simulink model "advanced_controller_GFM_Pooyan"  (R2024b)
settings: Solver=VariableStepAuto  StartTime=0.0  StopTime=2  RelTol=1e-3
model workspace (MAT data in the model file):
  b1 = 1000.38104695
  b2 = 1006.47399607
  b3 = 1006.95432939
  b4 = 996.322108769
  b5 = 995.669039411
  b6 = 1012.96535236
  b7 = 1007.5422409
  b8 = 993.960341463
  l1 = 8282.83466164
  l10 = 5511.54621883
  l11 = 8516.9845943
  l12 = 3533.51403234
  l13 = 1255.67117866
  l14 = 1105.23671469
  l15 = 955.492069576
  l16 = 1255.83166019
  l2 = 7767.51754481
  l3 = 6680.69860842
  l4 = 3013.93364227
  l5 = 912.604633733
  l6 = 706.803488619
  l7 = 1117.39027011
  l8 = 1674.30810947
  l9 = 1971.00014576
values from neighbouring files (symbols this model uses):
  alpha_p = 0.0001    [initialcondition_Pooyan.m]    (also in initialcondition_gfm_Pooyan.m = 0.0005)
  alpha_q = 0.0001    [initialcondition_Pooyan.m]    (also in initialcondition_gfm_Pooyan.m)
  Cf = 50e-6    (= 5e-05)    [initialcondition_Pooyan.m]    (also in initialcondition_gfm_Pooyan.m)
  Kicc = 314.159    [initialcondition_Pooyan.m]    (also in initialcondition_gfm_Pooyan.m)
  Kivc = 400    [initialcondition_Pooyan.m]    (also in initialcondition_gfm_Pooyan.m)
  Kpcc = 31.4159    [initialcondition_Pooyan.m]    (also in initialcondition_gfm_Pooyan.m)
  Kpvc = 0.5    [initialcondition_Pooyan.m]    (also in initialcondition_gfm_Pooyan.m)
  Lf = 10e-3    (= 0.01)    [initialcondition_Pooyan.m]    (also in initialcondition_gfm_Pooyan.m)
  Lg = X_BY_R*Rg/(wn)    [initialcondition_Pooyan.m]    (also in initialcondition_gfm_Pooyan.m; DER_param.m = (X_BY_R_gfl * Rg) / wn_gfl)
  Pn = 20e3    (= 20000)    [initialcondition_Pooyan.m]    (also in initialcondition_gfm_Pooyan.m)
  Qn = 0    [initialcondition_Pooyan.m]    (also in initialcondition_gfm_Pooyan.m)
  R = (3*Vg^2)/(2*Pn)    (= 8.000067)    [initialcondition_Pooyan.m]    (also in MC2.m = (8760*SS-sum(Tdown))/(8760*SS); initialcondition_gfm_Pooyan.m)
  Rf = 0.1    [initialcondition_Pooyan.m]    (also in initialcondition_gfm_Pooyan.m)
  Rg = (3*Vg^2)/(2*SCR*sqrt(1+X_BY_R^2)*Pn)    [initialcondition_Pooyan.m]    (also in initialcondition_gfm_Pooyan.m; DER_param.m = (3 * Vg_gfl^2) / (2 * SCR_gfl * sqrt(1 + X_BY_R_gfl^2) * Pn_)
  tau_p = 0.031415    [initialcondition_Pooyan.m]    (also in initialcondition_gfm_Pooyan.m)
  tau_q = 0.031415    [initialcondition_Pooyan.m]    (also in initialcondition_gfm_Pooyan.m)
  Ts = 50e-6    (= 5e-05)    [initialcondition_Pooyan.m]    (also in initialcondition_gfm_Pooyan.m)
  Vdc = 700    [initialcondition_Pooyan.m]    (also in initialcondition_gfm_Pooyan.m)
  Vg = 326.6    [initialcondition_Pooyan.m]    (also in initialcondition_gfm_Pooyan.m)
  wn = 2*pi*50    (= 314.159265359)    [initialcondition_Pooyan.m]    (also in initialcondition_gfm_Pooyan.m)
undefined symbols (not defined in the file or in its folder): DiscIntNeverNeededParam
libraries: simulink x8, spsThreePhaseSeriesRLCBranchLib x4, spsThreePhaseVIMeasurementLib x3, spsabctodq0Lib x3, spsGroundLib x2, spsDCVoltageSourceLib x1, spsThreePhaseSourceLib x1, spsThreePhaseBreakerLib x1, spsUniversalBridgeLib x1, spsdq0toabcLib x1, sps_lib x1

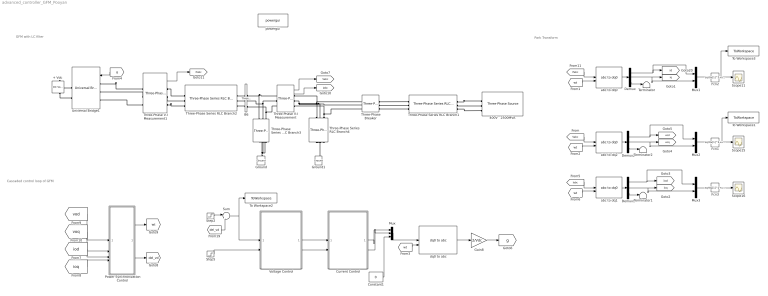
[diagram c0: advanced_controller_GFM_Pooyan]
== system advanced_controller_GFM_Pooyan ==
  note: Cascaded control loop of GFM
  note: GFM with LC filter
  note: Park Transform
  "+ Vdc " : spsDCVoltageSourceLib/DC Voltage Source  Amplitude=Vdc  Measurements=None
  400V   2500MVA : spsThreePhaseSourceLib/Three-Phase Source  InternalConnection=Yg  VoltagePhases=off  Voltage=Vg*sqrt(3/2)  PhaseAngle=0  Voltage_phases=[25e3 25e3 25e3]/sqrt(3)  PhaseAngles_phases=[0 -120 +120]  Frequency=50  NonIdealSource=on  SpecifyImpedance=off  Resistance=0  Inductance=0  ShortCircuitLevel=2500e6  BaseVoltage=Vg*sqrt(3/2)  XRratio=7  BusType=swing  Pref=0  Qref=0  Prefabc=[10e3, 10e3, 10e3]  Qrefabc=[0, 0, 0]  Qmin=-inf  Qmax=inf
  B6 : spsThreePhaseVIMeasurementLib/Three-Phase V-I Measurement  VoltageMeasurement=phase-to-ground  SetLabelV=on  LabelV=Vabcg  Vpu=on  VpuLL=off  CurrentMeasurement=yes  SetLabelI=on  LabelI=Iabcg  Ipu=off  Pbase=100e3  Vbase=415  OutputType=Magnitude  PhasorSimulation=off  PSBequivalent=0
  Constant1 : Constant  Value=0
  Current Control : Subsystem
  Demux : Demux  Outputs=3
  Demux1 : Demux  Outputs=3
  Demux2 : Demux  Outputs=3
  Fcn1 : Fcn  Expr=sqrt(u[1]^2+u[2]^2)
  Fcn2 : Fcn  Expr=sqrt(u[1]^2+u[2]^2)
  Fcn3 : Fcn  Expr=sqrt(u[1]^2+u[2]^2)
  Gain8 : Gain  Gain=2/Vdc
  Ground : spsGroundLib/Ground  LConnTagsString=a
  Ground1 : spsGroundLib/Ground  LConnTagsString=a
  Mux : Mux  Inputs=3
  Mux1 : Mux  Inputs=2
  Mux2 : Mux  Inputs=2
  Mux3 : Mux  Inputs=2
  Power Synchronization Control : Subsystem
  Scope11 : Scope
  Scope15 : Scope
  Scope16 : Scope
  Step2 : Step  Time=100  Before=Vg  After=Vg  SampleTime=0
  Step5 : Step  Time=100  After=0  SampleTime=0
  Sum : Sum  Inputs=|++
  Terminator : Terminator
  Terminator1 : Terminator
  Terminator2 : Terminator
  Three-Phase Series RLC Branch1 : spsThreePhaseSeriesRLCBranchLib/Three-Phase Series RLC Branch  LConnTagsString=A|B|C  RConnTagsString=A|B|C  BranchType=RL  Resistance=Rg  Inductance=Lg  Capacitance=1e-6  Measurements=None
  Three-Phase Series RLC Branch2 : spsThreePhaseSeriesRLCBranchLib/Three-Phase Series RLC Branch  LConnTagsString=A|B|C  RConnTagsString=A|B|C  BranchType=RL  Resistance=Rf  Inductance=Lf  Capacitance=1e-6  Measurements=None
  Three-Phase Series RLC Branch3 : spsThreePhaseSeriesRLCBranchLib/Three-Phase Series RLC Branch  LConnTagsString=A|B|C  RConnTagsString=A|B|C  BranchType=C  Resistance=0.1  Inductance=280e-3  Capacitance=Cf  Measurements=None
  Three-Phase Series RLC Branch4 : spsThreePhaseSeriesRLCBranchLib/Three-Phase Series RLC Branch  LConnTagsString=A|B|C  RConnTagsString=A|B|C  BranchType=R  Resistance=R  Inductance=0  Capacitance=1e-6  Measurements=None
  Three-Phase V-I Measurement : spsThreePhaseVIMeasurementLib/Three-Phase V-I Measurement  VoltageMeasurement=phase-to-ground  SetLabelV=off  LabelV=Vabc  Vpu=off  VpuLL=off  CurrentMeasurement=yes  SetLabelI=off  LabelI=Iabc  Ipu=off  Pbase=100e6  Vbase=500e3  OutputType=Complex  PhasorSimulation=off  PSBequivalent=0
  Three-Phase V-I Measurement1 : spsThreePhaseVIMeasurementLib/Three-Phase V-I Measurement  VoltageMeasurement=no  SetLabelV=off  LabelV=Vabc  Vpu=off  VpuLL=off  CurrentMeasurement=yes  SetLabelI=off  LabelI=Iabc  Ipu=off  Pbase=100e6  Vbase=500e3  OutputType=Complex  PhasorSimulation=off  PSBequivalent=0
  Three-Phase Breaker : spsThreePhaseBreakerLib/Three-Phase Breaker  InitialState=open  SwitchA=on  SwitchB=on  SwitchC=on  SwitchTimes=[0.5]  External=off  BreakerResistance=0.01  SnubberResistance=1e6  SnubberCapacitance=inf  Measurements=None
  To Workspace1 : ToWorkspace  VariableName=vo2  SampleTime=-1
  To Workspace2 : ToWorkspace  VariableName=vd_ref  SampleTime=-1
  To Workspace3 : ToWorkspace  VariableName=if2  SampleTime=-1
  Universal Bridge1 : spsUniversalBridgeLib/Universal Bridge  Arms=3  SnubberResistance=1e5  SnubberCapacitance=inf  Device=Average-model based VSC  Ron=1e-3  Lon=0  ForwardVoltages="[  0  0  ]"  ForwardVoltage=0  GTOparameters=[ 10e-6 , 20e-6 ]  IGBTparameters=[ 1e-6 , 2e-6 ]  Measurements=None  Measurements_2=None  converterType=Rectifier
  Voltage Control : Subsystem
  abc to dq0 : spsabctodq0Lib/abc to dq0  Alignment=90 degrees behind phase A axis
  abc to dq1 : spsabctodq0Lib/abc to dq0  Alignment=90 degrees behind phase A axis
  abc to dq2 : spsabctodq0Lib/abc to dq0  Alignment=90 degrees behind phase A axis
  dq0 to abc : spsdq0toabcLib/dq0 to abc  Alignment=90 degrees behind phase A axis
  powergui : sps_lib/powergui  Priority=1  SimulationMode=Discrete  SampleTime=Ts  frequency=50  Iterations=50  frequencyindice=0  Pbase=100e6  ErrMax=1e-4  UnitsV=kV  UnitsW=MW  buscounter=0  FunctionMessages=off  echomessages=off  EnableUseOfTLC=off  CurrentSourceSwitches=off  DisableSnubberDevices=off  DisableRonSwitches=off  DisableVfSwitches=off  DisplayEquations=off  AutomaticDiscreteSolvers=off  SolverType=Tustin  Interpol=off  ExternalGateDelay=off  methode=off  Ts=0  x0status=blocks  SPID=off  SwTol=0  HookPort=off  NonlinearTolerance=0  nMaxIteration=15  ContinueOnMaxIteration=off  RestoreLinks=warning  ResistiveCurrentMeasurement=off  Frange=[0:2:500]  Ylog=off  Xlog=on  ShowGrid=off  save=off  variable=ZData  structure=0  ZoomFFT=on  StartTime=0.0  cycles=1  DisplayStyle=1  fundamental=60  FreqAxis=off  MaxFrequency=1000  frequencyindicesteady=1  RmsSteady=1  display=off
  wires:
  Gain8/1 -> [g]
  Demux/3 -> Terminator/1
  abc to dq1/1 -> Demux1/1
  Step2/1 -> Sum/1
  [wt] -> dq0 to abc/2
  Constant1/1 -> Mux/3
  [ioq] -> Power Synchronization Control/4(In4)
  [iod] -> Power Synchronization Control/3(In3)
  dq0 to abc/1 -> Gain8/1
  Demux/2 -> Mux1/2, [iq]
  Mux/1 -> dq0 to abc/1
  [wt] -> abc to dq2/2
  [vod] -> Power Synchronization Control/1(In1)
  Demux1/3 -> Terminator1/1
  Demux1/2 -> Mux3/2, [ioq]
  Voltage Control/2(iqref) -> Current Control/2(iqref)
  Current Control/2(vqt) -> Mux/2
  [voq] -> Power Synchronization Control/2(In2)
  Demux1/1 -> Mux3/1, [iod]
  Demux2/1 -> Mux2/1, [vod]
  [g] -> Universal Bridge1/1
  [del_vd] -> Sum/2
  Voltage Control/1(idref) -> Current Control/1(idref)
  [wt] -> abc to dq0/2
  Demux/1 -> Mux1/1, [id]
  abc to dq2/1 -> Demux2/1
  Current Control/1(vdt) -> Mux/1
  Demux2/3 -> Terminator2/1
  Power Synchronization Control/2(del_vd) -> [del_vd]
  Sum/1 -> Voltage Control/1(vodref), To Workspace2/1
  Power Synchronization Control/1(wt) -> [wt]
  Demux2/2 -> [voq], Mux2/2
  abc to dq0/1 -> Demux/1
  Mux1/1 -> Fcn2/1
  Fcn2/1 -> To Workspace3/1, Scope11/1
  Mux2/1 -> Fcn1/1
  Fcn1/1 -> To Workspace1/1, Scope15/1
  Fcn3/1 -> Scope16/1
  Mux3/1 -> Fcn3/1
  Three-Phase V-I Measurement/1 -> [Vabc]
  [Vabc] -> abc to dq2/1
  Three-Phase V-I Measurement/2 -> [Iabc]
  [Iabc] -> abc to dq1/1
  [wt] -> abc to dq1/2
  Three-Phase V-I Measurement1/1 -> [Ifabc]
  [Ifabc] -> abc to dq0/1
  Step5/1 -> Voltage Control/2(voqref)
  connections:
  Three-Phase Series RLC Branch3/LConn3 -- Three-Phase V-I Measurement/LConn3 -- B6/RConn3
  Three-Phase Series RLC Branch4/LConn1 -- Three-Phase Breaker/LConn1 -- Three-Phase V-I Measurement/RConn1
  Three-Phase Series RLC Branch3/LConn1 -- Three-Phase V-I Measurement/LConn1 -- B6/RConn1
  Three-Phase Series RLC Branch4/RConn3 -- Three-Phase Series RLC Branch4/RConn1 -- Ground1/LConn1 -- Three-Phase Series RLC Branch4/RConn2
  Three-Phase V-I Measurement/RConn2 -- Three-Phase Breaker/LConn2 -- Three-Phase Series RLC Branch4/LConn2
  Three-Phase Series RLC Branch3/LConn2 -- B6/RConn2 -- Three-Phase V-I Measurement/LConn2
  Ground/LConn1 -- Three-Phase Series RLC Branch3/RConn1 -- Three-Phase Series RLC Branch3/RConn2 -- Three-Phase Series RLC Branch3/RConn3
  Three-Phase Series RLC Branch4/LConn3 -- Three-Phase Breaker/LConn3 -- Three-Phase V-I Measurement/RConn3
  Three-Phase V-I Measurement1/LConn3 -- Universal Bridge1/LConn3
  Three-Phase V-I Measurement1/LConn2 -- Universal Bridge1/LConn2
  Three-Phase Breaker/RConn1 -- Three-Phase Series RLC Branch1/LConn1
  Three-Phase Breaker/RConn3 -- Three-Phase Series RLC Branch1/LConn3
  Three-Phase Series RLC Branch1/RConn1 -- 400V   2500MVA/RConn1
  Three-Phase V-I Measurement1/RConn1 -- Three-Phase Series RLC Branch2/LConn1
  "+ Vdc "/RConn1 -- Universal Bridge1/RConn1
  Three-Phase Series RLC Branch1/RConn2 -- 400V   2500MVA/RConn2
  Three-Phase Series RLC Branch1/RConn3 -- 400V   2500MVA/RConn3
  "+ Vdc "/LConn1 -- Universal Bridge1/RConn2
  Three-Phase Breaker/RConn2 -- Three-Phase Series RLC Branch1/LConn2
  Three-Phase V-I Measurement1/RConn2 -- Three-Phase Series RLC Branch2/LConn2
  Universal Bridge1/LConn1 -- Three-Phase V-I Measurement1/LConn1
  B6/LConn3 -- Three-Phase Series RLC Branch2/RConn3
  B6/LConn2 -- Three-Phase Series RLC Branch2/RConn2
  Three-Phase V-I Measurement1/RConn3 -- Three-Phase Series RLC Branch2/LConn3
  B6/LConn1 -- Three-Phase Series RLC Branch2/RConn1

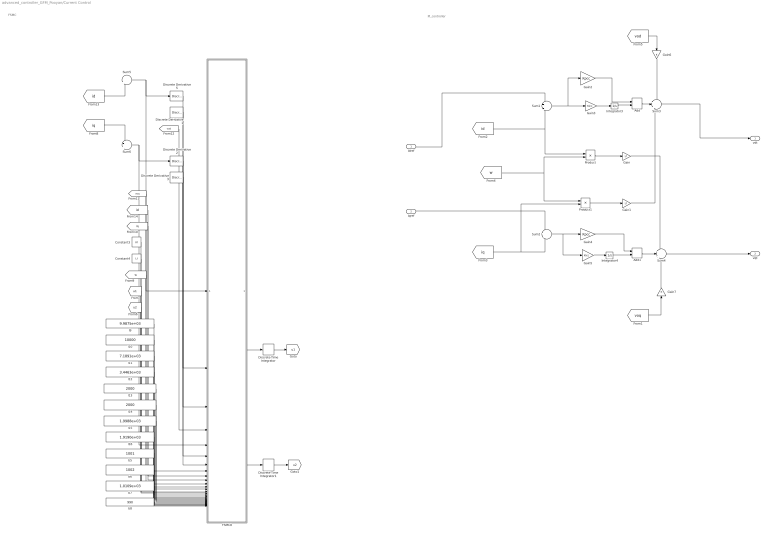
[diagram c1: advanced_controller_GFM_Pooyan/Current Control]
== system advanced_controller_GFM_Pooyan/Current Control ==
  note: PI_controller
  note: FSMC
  idref : Inport
  iqref : Inport  Port=2
  Add : Sum
  Add1 : Sum
  Constant3 : Constant  Commented=on  Value=Rf
  Constant4 : Constant  Commented=on  Value=Lf
  Discrete Derivative{1..3,5} (4 alike) : simulink/Quick Insert/Discrete/Discrete Derivative  Commented=on  gainval=1.0  ICPrevScaledInput=0.0  OutMin=[]  OutMax=[]  OutDataType=fixdt(1, 16)  OutScaling=2^-10  DoSatur=off
  Discrete-Time Integrator : DiscreteIntegrator  Commented=on  SampleTime=-1  ICPrevOutput=DiscIntNeverNeededParam  ICPrevScaledInput=DiscIntNeverNeededParam
  Discrete-Time Integrator1 : DiscreteIntegrator  Commented=on  SampleTime=-1  ICPrevOutput=DiscIntNeverNeededParam  ICPrevScaledInput=DiscIntNeverNeededParam
  FSMC8 : MATLAB Function  Commented=on  TreatAsAtomicUnit=on
  Gain : Gain  Gain=Lf
  Gain1 : Gain  Gain=Lf
  Gain2 : Gain  Gain=Kpcc
  Gain3 : Gain  Gain=Kicc
  Gain4 : Gain  Gain=Kpcc
  Gain5 : Gain  Gain=Kicc
  Gain6 : Gain
  Gain7 : Gain
  Integrator3 : Integrator
  Integrator4 : Integrator
  Product : Product
  Product1 : Product
  Sum1 : Sum  Inputs=+|-
  Sum2 : Sum  Inputs=+|-
  Sum3 : Sum  Inputs=+|+|-
  Sum4 : Sum  Inputs=+|+|+
  Sum5 : Sum  Commented=on  Inputs=|+-
  Sum6 : Sum  Commented=on  Inputs=-+|
  b5 : Constant  Commented=on  Value=1001
  b6 : Constant  Commented=on  Value=1002
  b7 : Constant  Commented=on  Value=1.0109e+03
  b8 : Constant  Commented=on  Value=990
  l10 : Constant  Commented=on  Value=10000
  l11 : Constant  Commented=on  Value=7.1891e+03
  l12 : Constant  Commented=on  Value=3.4463e+03
  l13 : Constant  Commented=on  Value=2000
  l14 : Constant  Commented=on  Value=2000
  l15 : Constant  Commented=on  Value=1.9988e+03
  l16 : Constant  Commented=on  Value=1.9190e+03
  l9 : Constant  Commented=on  Value=9.9875e+03
  vdt : Outport
  vqt : Outport  Port=2
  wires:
  Gain3/1 -> Integrator3/1
  Integrator4/1 -> Add1/2
  Add/1 -> Sum3/2
  Gain4/1 -> Add1/1
  Add1/1 -> Sum4/2
  Gain2/1 -> Add/1
  Gain/1 -> Sum4/1
  Gain1/1 -> Sum3/3
  Integrator3/1 -> Add/2
  Gain5/1 -> Integrator4/1
  iqref/1 -> Sum2/1
  [iq] -> Sum2/2, Product1/2
  idref/1 -> Sum1/1
  [id] -> Product/1, Sum1/2
  Product/1 -> Gain/1
  Product1/1 -> Gain1/1
  [w] -> Product1/1, Product/2
  [vod] -> Gain6/1
  [voq] -> Gain7/1
  Gain6/1 -> Sum3/1
  Gain7/1 -> Sum4/3
  Sum3/1 -> vdt/1
  Sum4/1 -> vqt/1
  Constant4/1 -> FSMC8/12(Lf)
  l10/1 -> FSMC8/17(a_2)
  Discrete Derivative2/1 -> FSMC8/6(e2dot)
  b7/1 -> FSMC8/26(betta2s)
  FSMC8/2(vqt) -> ?
  FSMC8/3(u1dot) -> Discrete-Time Integrator/1
  Discrete Derivative5/1 -> FSMC8/2(e1dot)
  [w] -> FSMC8/13(w)
  Sum6/1 -> FSMC8/5(e2), Discrete Derivative2/1
  Sum5/1 -> FSMC8/1(e1), Discrete Derivative5/1
  [voq] -> FSMC8/8(voq)
  Constant3/1 -> FSMC8/11(Rf)
  l16/1 -> FSMC8/23(a_8)
  [iq] -> FSMC8/10(ioq)
  l13/1 -> FSMC8/20(a_5)
  l11/1 -> FSMC8/18(a_3)
  [id] -> Sum5/2
  FSMC8/1(vdt) -> ?
  b6/1 -> FSMC8/25(betta1m)
  l12/1 -> FSMC8/19(a_4)
  l14/1 -> FSMC8/21(a_6)
  Discrete Derivative3/1 -> FSMC8/7(iqrefdot)
  b5/1 -> FSMC8/24(betta1s)
  l9/1 -> FSMC8/16(a_1)
  b8/1 -> FSMC8/27(betta2m)
  [id] -> FSMC8/9(iod)
  Discrete Derivative1/1 -> FSMC8/3(idrefdot)
  FSMC8/4(u2dot) -> Discrete-Time Integrator1/1
  ? -> Discrete Derivative1/1, Sum5/1
  [vod] -> FSMC8/4(vod)
  [iq] -> Sum6/1
  ? -> Discrete Derivative3/1, Sum6/2
  l15/1 -> FSMC8/22(a_7)
  Sum1/1 -> Gain3/1, Gain2/1
  Sum2/1 -> Gain5/1, Gain4/1
  Discrete-Time Integrator/1 -> [u1]
  Discrete-Time Integrator1/1 -> [u2]
  [u1] -> FSMC8/14(u1)
  [u2] -> FSMC8/15(u2)

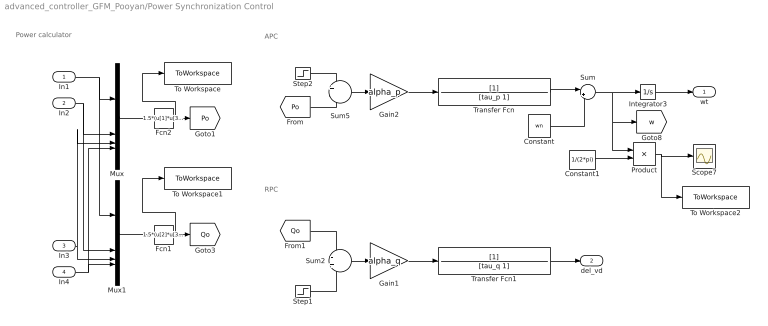
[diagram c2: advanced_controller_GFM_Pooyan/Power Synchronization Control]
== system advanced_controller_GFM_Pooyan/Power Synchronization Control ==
  note: APC
  note: RPC
  note: Power calculator
  In1 : Inport
  In2 : Inport  Port=2
  In3 : Inport  Port=3
  In4 : Inport  Port=4
  Constant : Constant  Value=wn
  Constant1 : Constant  Value=1/(2*pi)
  Fcn1 : Fcn  Expr=1.5*(u[2]*u[3]-u[1]*u[4])
  Fcn2 : Fcn  Expr=1.5*(u[1]*u[3]+u[2]*u[4])
  Gain1 : Gain  Gain=alpha_q
  Gain2 : Gain  Gain=alpha_p
  Integrator3 : Integrator
  Mux : Mux
  Mux1 : Mux
  Product : Product
  Scope7 : Scope
  Step1 : Step  Time=100  Before=Qn  After=Qn  SampleTime=0
  Step2 : Step  Time=100  Before=Pn  After=Pn  SampleTime=0
  Sum : Sum  Inputs=|++
  Sum2 : Sum  Inputs=-+
  Sum5 : Sum  Inputs=+-
  To Workspace : ToWorkspace  VariableName=Po  SampleTime=-1
  To Workspace1 : ToWorkspace  VariableName=Qo  SampleTime=-1
  To Workspace2 : ToWorkspace  VariableName=f  SampleTime=-1
  Transfer Fcn : TransferFcn  Denominator=[tau_p 1]  ParameterTunability=Unconstrained
  Transfer Fcn1 : TransferFcn  Denominator=[tau_q 1]  ParameterTunability=Unconstrained
  wt : Outport
  del_vd : Outport  Port=2
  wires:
  Sum5/1 -> Gain2/1
  [Po] -> Sum5/2
  Fcn2/1 -> To Workspace/1, [Po]
  [Qo] -> Sum2/1
  Step1/1 -> Sum2/2
  Sum2/1 -> Gain1/1
  Step2/1 -> Sum5/1
  Gain1/1 -> Transfer Fcn1/1
  Transfer Fcn1/1 -> del_vd/1
  Gain2/1 -> Transfer Fcn/1
  Transfer Fcn/1 -> Sum/1
  Constant/1 -> Sum/2
  Sum/1 -> [w], Product/1, Integrator3/1
  Mux/1 -> Fcn2/1
  Constant1/1 -> Product/2
  Integrator3/1 -> wt/1
  Product/1 -> To Workspace2/1, Scope7/1
  In3/1 -> Mux1/3, Mux/3
  In1/1 -> Mux1/1, Mux/1
  In4/1 -> Mux/4, Mux1/4
  In2/1 -> Mux1/2, Mux/2
  Mux1/1 -> Fcn1/1
  Fcn1/1 -> To Workspace1/1, [Qo]

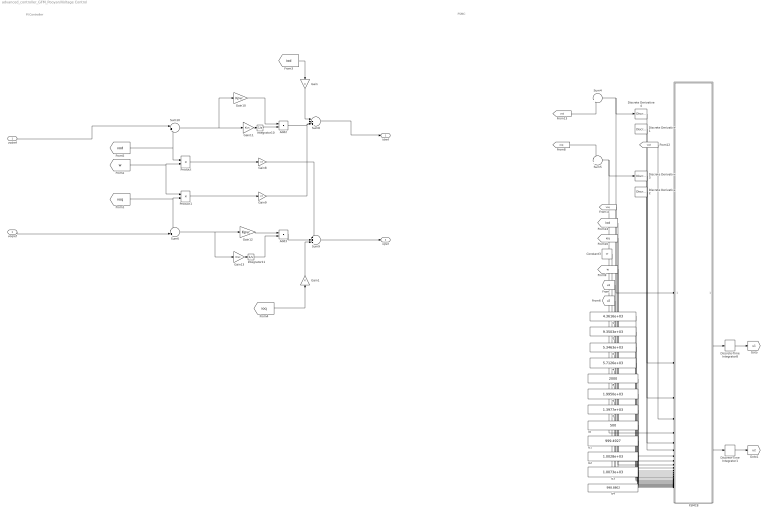
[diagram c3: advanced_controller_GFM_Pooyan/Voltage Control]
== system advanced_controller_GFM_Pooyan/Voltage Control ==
  note: PI Controller
  note: FSMC
  vodref : Inport
  voqref : Inport  Port=2
  Add2 : Sum
  Add3 : Sum
  Constant3 : Constant  Commented=on  Value=Cf
  Discrete Derivative{1..4} (4 alike) : simulink/Quick Insert/Discrete/Discrete Derivative  Commented=on  gainval=1.0  ICPrevScaledInput=0.0  OutMin=[]  OutMax=[]  OutDataType=fixdt(1, 16)  OutScaling=2^-10  DoSatur=off
  Discrete-Time Integrator1 : DiscreteIntegrator  Commented=on  SampleTime=-1  ICPrevOutput=DiscIntNeverNeededParam  ICPrevScaledInput=DiscIntNeverNeededParam
  Discrete-Time Integrator8 : DiscreteIntegrator  Commented=on  SampleTime=-1  ICPrevOutput=DiscIntNeverNeededParam  ICPrevScaledInput=DiscIntNeverNeededParam
  FSMC8 : MATLAB Function  Commented=on  TreatAsAtomicUnit=on
  Gain : Gain
  Gain1 : Gain
  Gain10 : Gain  Gain=Kpvc
  Gain11 : Gain  Gain=Kivc
  Gain12 : Gain  Gain=Kpvc
  Gain13 : Gain  Gain=Kivc
  Gain8 : Gain  Gain=Cf
  Gain9 : Gain  Gain=Cf
  Integrator10 : Integrator
  Integrator11 : Integrator
  Product : Product
  Product1 : Product
  Sum10 : Sum  Inputs=|+-
  Sum4 : Sum  Commented=on  Inputs=|+-
  Sum5 : Sum  Commented=on  Inputs=-+|
  Sum6 : Sum  Inputs=-+|
  Sum8 : Sum  Inputs=|++-
  Sum9 : Sum  Inputs=+++|
  b1 : Constant  Commented=on  Value=999.4927
  b2 : Constant  Commented=on  Value=1.0028e+03
  b3 : Constant  Commented=on  Value=1.0073e+03
  b4 : Constant  Commented=on  Value=998.8802
  l1 : Constant  Commented=on  Value=4.3616e+03
  l2 : Constant  Commented=on  Value=9.3503e+03
  l3 : Constant  Commented=on  Value=5.3463e+03
  l4 : Constant  Commented=on  Value=5.7126e+03
  l5 : Constant  Commented=on  Value=2000
  l6 : Constant  Commented=on  Value=1.9950e+03
  l7 : Constant  Commented=on  Value=1.3977e+03
  l8 : Constant  Commented=on  Value=500
  idref : Outport
  iqref : Outport  Port=2
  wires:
  Gain12/1 -> Add3/1
  voqref/1 -> Sum6/2
  Gain13/1 -> Integrator11/1
  Gain8/1 -> Sum9/1
  [vod] -> Sum10/2, Product/1
  [voq] -> Product1/2, Sum6/1
  Integrator11/1 -> Add3/2
  Gain11/1 -> Integrator10/1
  Gain10/1 -> Add2/1
  Add3/1 -> Sum9/2
  Integrator10/1 -> Add2/2
  vodref/1 -> Sum10/1
  [w] -> Product/2, Product1/1
  Product/1 -> Gain8/1
  Product1/1 -> Gain9/1
  Sum8/1 -> idref/1
  Sum9/1 -> iqref/1
  Add2/1 -> Sum8/2
  Gain9/1 -> Sum8/3
  [iod] -> Gain/1
  Gain/1 -> Sum8/1
  [ioq] -> Gain1/1
  Gain1/1 -> Sum9/3
  FSMC8/2(iqref) -> ?
  FSMC8/1(idref) -> ?
  ? -> Sum5/2, Discrete Derivative2/1
  [w] -> FSMC8/12(w)
  [vod] -> FSMC8/4(vod)
  Discrete Derivative3/1 -> FSMC8/6(e2dot)
  Discrete Derivative4/1 -> FSMC8/2(e1dot)
  l7/1 -> FSMC8/21(a7)
  FSMC8/3(u1dot) -> Discrete-Time Integrator8/1
  b4/1 -> FSMC8/26(betta2m)
  Sum4/1 -> Discrete Derivative4/1, FSMC8/1(e1)
  b3/1 -> FSMC8/25(betta2s)
  FSMC8/4(u2dot) -> Discrete-Time Integrator1/1
  l8/1 -> FSMC8/22(a8)
  l1/1 -> FSMC8/15(a1)
  b2/1 -> FSMC8/24(betta1m)
  [vod] -> Sum4/2
  l6/1 -> FSMC8/20(a6)
  l3/1 -> FSMC8/17(a3)
  Discrete Derivative2/1 -> FSMC8/7(dvoqref)
  Sum5/1 -> FSMC8/5(e2), Discrete Derivative3/1
  l5/1 -> FSMC8/19(a5)
  l4/1 -> FSMC8/18(a4)
  Discrete Derivative1/1 -> FSMC8/3(dvodref)
  [voq] -> Sum5/1
  [iod] -> FSMC8/9(iod)
  l2/1 -> FSMC8/16(a2)
  [ioq] -> FSMC8/10(ioq)
  b1/1 -> FSMC8/23(betta1s)
  Constant3/1 -> FSMC8/11(Cf)
  [voq] -> FSMC8/8(voq)
  ? -> Discrete Derivative1/1, Sum4/1
  Sum10/1 -> Gain10/1, Gain11/1
  Sum6/1 -> Gain12/1, Gain13/1
  Discrete-Time Integrator1/1 -> [u2]
  Discrete-Time Integrator8/1 -> [u1]
  [u1] -> FSMC8/13(u1)
  [u2] -> FSMC8/14(u2)

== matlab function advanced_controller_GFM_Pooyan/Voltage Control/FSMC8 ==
function [idref,iqref,u1dot,u2dot]= fcn(e1,e1dot,dvodref,vod,e2,e2dot,dvoqref,voq,iod,ioq,Cf,w,u1,u2,a1,a2,a3,a4,a5,a6,a7,a8,betta1s,betta1m,betta2s,betta2m)

sig3=((nthroot(abs(e1),betta1m))^betta1s)*sign(e1);
sig4=((nthroot(abs(e1),betta2m))^betta2s)*sign(e1);
A1=a1*sig3;
B1=a2*sig4;
s1=e1dot+A1+B1;

sig33=((nthroot(abs(e2),betta1m))^betta1s)*sign(e2);
sig44=((nthroot(abs(e2),betta2m))^betta2s)*sign(e2);
A2=a3*sig33;
B2=a4*sig44;
s2=e2dot+A2+B2;

%controller
sig1=((nthroot(abs(s1),betta1m))^betta1s)*sign(s1);
sig2=((nthroot(abs(s1),betta2m))^betta2s)*sign(s1);
u1dot=a5*sig1+a6*sig2;
idref=(Cf)*(iod/Cf-w*voq+A1+B1+u1+dvodref);

sig11=((nthroot(abs(s2),betta1m))^betta1s)*sign(s2);
sig22=((nthroot(abs(s2),betta2m))^betta2s)*sign(s2);

u2dot=a7*sig11+a8*sig22;
iqref=(Cf)*(ioq/Cf+w*vod+A2+B2+u2+dvoqref);

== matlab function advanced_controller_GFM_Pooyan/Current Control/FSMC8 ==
function [vdt,vqt,u1dot,u2dot]= fcn(e1,e1dot,idrefdot,vod,e2,e2dot,iqrefdot,voq,iod,ioq,Rf,Lf,w,u1,u2,a_1,a_2,a_3,a_4,a_5,a_6,a_7,a_8,betta1s,betta1m,betta2s,betta2m)

sig3=((nthroot(abs(e1),betta1m))^betta1s)*sign(e1);
sig4=((nthroot(abs(e1),betta2m))^betta2s)*sign(e1);
A1=a_1*sig3;
B1=a_2*sig4;
s1=e1dot+A1+B1;

sig33=((nthroot(abs(e2),betta1m))^betta1s)*sign(e2);
sig44=((nthroot(abs(e2),betta2m))^betta2s)*sign(e2);
A2=a_3*sig33;
B2=a_4*sig44;
s2=e2dot+A2+B2;

%controller
sig1=((nthroot(abs(s1),betta1m))^betta1s)*sign(s1);
sig2=((nthroot(abs(s1),betta2m))^betta2s)*sign(s1);

u1dot=a_5*sig1+a_6*sig2;
vdt=(Lf)*(vod/Lf+Rf*iod/Lf-w*ioq+A1+B1+u1+idrefdot);

sig11=((nthroot(abs(s2),betta1m))^betta1s)*sign(s2);
sig22=((nthroot(abs(s2),betta2m))^betta2s)*sign(s2);

u2dot=a_7*sig11+a_8*sig22;
vqt=(Lf)*(voq/Lf+Rf*ioq/Lf+w*iod+A2+B2+u2+iqrefdot);
